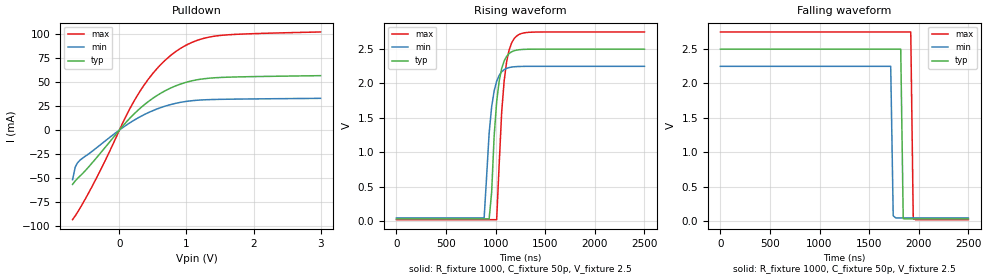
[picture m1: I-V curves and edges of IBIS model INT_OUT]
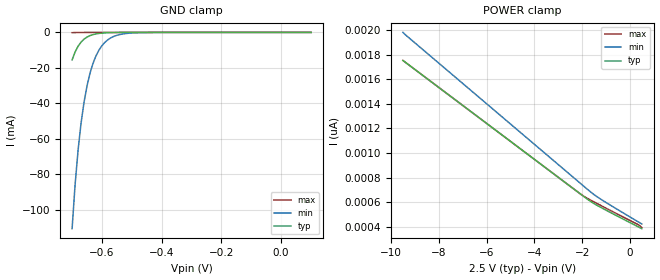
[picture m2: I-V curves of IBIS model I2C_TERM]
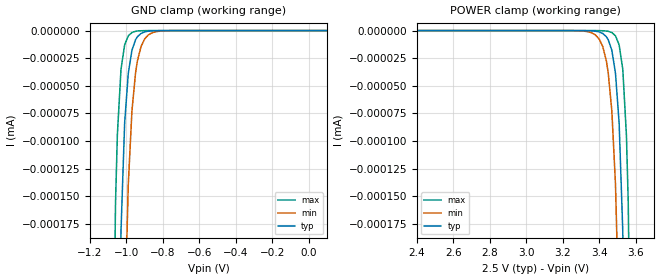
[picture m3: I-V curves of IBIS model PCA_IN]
|   NXP Semiconductors Inc.
|   Specialty Logic Products Group
|   IBIS model of PCA9544A
|   4-Channel I2C switch with
|   interrupt logic
[IBIS Ver]   3.2
[Comment Char]   |_char
| VDD typ = 2.5V, min = 2.25V and max = 2.75V
[File name]   pca9544a_2_5v.ibs
[File Rev]   1.0
[Date]   Nov 29, 2007 11:15:22 AM
[Source]
Generated by Seshadri Venkataramanan with IbisToolKit at Tempe, AZ
[Notes]
[Disclaimer]
* All rights reserved
NXP Semiconductors warrants and represents that the IBIS models identified
herein are owned by NXP Semiconductors (NXP). The
models provided are not warranted as fully representing all of the operating
characteristics and specifications of the semiconductor products to which the
models relate. Moreover, unless there is a
signed, written agreement to the contrary, these models are furnished on an "as
is" basis without support or warranty of any kind, either expressed or implied,
regarding the use thereof, and NXP specifically disclaims all implied warranties
of merchantability and
fitness of the models for any purpose.
NXP does not assume any liability arising out of the application or use of these
IBIS models including infringement of patents and
copyrights, nor does NXP convey any license under its patents and copyrights or
the rights of others.
NXP provides IBIS models as a service to our customers. You and your company
shall not distribute, convey, sell, or give these models
to anyone else without receiving prior written permission from NXP.(C) Copyright
2007 NXP Semiconductors
NXP Semiconductors (NXP) does not warrant that this model and any other
accompanying information (Model) accurately or fully represents the
operating characteristics and specifications of the semiconductor
products to which the Model relates.  Moreover, the Model is furnished
on an "as is" and with "all faults" basis, and without support or
warranty of any kind.  NXP disclaims all warranties, whether expressed
or implied or statutory, including without limitation all implied
warranties of non-infringement, merchantability and fitness for any
purpose, and those arising from a course of dealing or usage of trade.
NXP does not convey any license under its or any third party's patents,
copyrights or other intellectual property or proprietary rights.
You and your company assume any and all risks and liability arising out
of the application or use of the Model.
In no event shall NXP be liable for any direct, indirect, special,
consequential or incidental damages, however caused, whether in
warranty, contract or tort (including negligence), strict liability or
other legal theory, including, without limitation, for lost profits,
business interruption, or corruption or loss of data or information,
arising out of or in connection with the use of or the inability to use
the Model, even if NXP has been advised of the possibility of such
damages.
NXP provides the Model as a courtesy to our customers. You and your
company shall not distribute, convey, sell, or give the Model to anyone
else without receiving prior written permission from NXP.
NXP reserves the right to make changes without notice to the Model to
improve reliability, function, or design.
Please be aware that your receipt and subsequent use of the Model shall
serve as acceptance of these terms and conditions.  If you do not
accept these terms, return or destroy the Model immediately.
[Copyright]
2007
[Component]   PCA9544AD
Si_location Pin
Timing_location Pin
[Manufacturer]   NXP Semiconductors
[Package]
|   variable   typ   min   max
R_pkg   5.95E-02   5.36E-02   6.59E-02
L_pkg   4.21E-09   3.07E-09   5.91E-09
C_pkg   0.910E-12   0.758E-12   1.110E-12
|   SO20
[Pin] signal_name   model_name   R_pin   L_pin   C_pin
1   A0   PCA_IN   5.75E-02  5.91E-09  1.050E-12
2   A1   PCA_IN   6.25E-02  4.85E-09  1.040E-12
3   a2   PCA_IN   6.59E-02  3.92E-09  0.861E-12
4   INT0B   INT_IN   5.79E-02  3.32E-09  0.803E-12
5   SD0   I2C_TERM   5.36E-02  3.07E-09  0.758E-12
6   SC0   I2C_TERM   5.36E-02  3.07E-09  0.758E-12
7   INT1B   INT_IN   5.79E-02  3.32E-09  0.803E-12
8   SD1   I2C_TERM   6.59E-02  3.92E-09  0.861E-12
9   SC1   I2C_TERM   6.25E-02  4.85E-09  1.040E-12
10   Vss   GND   5.75E-02  5.91E-09  1.110E-12
11   INT2B   INT_IN   5.75E-02  5.91E-09  1.110E-12
12   SD2   I2C_TERM   6.25E-02  4.85E-09  1.040E-12
13   SC2   I2C_TERM   6.59E-02  3.92E-09  0.861E-12
14   INT3B   INT_IN   5.79E-02  3.32E-09  0.803E-12
15   SD3   I2C_TERM   5.36E-02  3.07E-09  0.758E-12
16   SC3   I2C_TERM   5.36E-02  3.07E-09  0.758E-12
17   INTB   INT_OUT   5.79E-02  3.32E-09  0.803E-12
18   SCL   I2C_TERM   6.59E-02  3.92E-09  0.861E-12
19   SDA   I2C_TERM   6.25E-02  4.85E-09  1.040E-12
20   Vdd   POWER   5.75E-02  5.91E-09  1.110E-12
[Component]   PCA9544APW
Si_location Pin
Timing_location Pin
[Manufacturer]   NXP Semiconductors
[Package]
|   variable   typ   min   max
R_pkg   7.24E-02   6.63E-02   8.34E-02
L_pkg   2.47E-09   2.09E-09   3.18E-09
C_pkg   0.341E-12   0.282E-12   0.420E-12
|   TSSOP20
[Pin] signal_name   model_name   R_pin   L_pin   C_pin
1   A0   PCA_IN   6.63E-02  3.18E-09  0.408E-12
2   A1   PCA_IN   6.67E-02  2.55E-09  0.398E-12
3   A2   PCA_IN   8.34E-02  2.35E-09  0.317E-12
4   INT0B   INT_IN   7.44E-02  2.16E-09  0.293E-12
5   SD0   I2C_TERM   7.10E-02  2.09E-09  0.282E-12
6   SC0   I2C_TERM   7.10E-02  2.09E-09  0.282E-12
7   INT1B   INT_IN   7.44E-02  2.16E-09  0.293E-12
8   SD1   I2C_TERM   8.34E-02  2.35E-09  0.317E-12
9   SC1   I2C_TERM   6.67E-02  2.55E-09  0.397E-12
10   Vss   GND   6.63E-02  3.18E-09  0.420E-12
11   INT2B   INT_IN   6.63E-02  3.17E-09  0.420E-12
12   SD2   I2C_TERM   6.67E-02  2.55E-09  0.397E-12
13   SC2   I2C_TERM   8.34E-02  2.35E-09  0.317E-12
14   INT3B   INT_IN   7.44E-02  2.16E-09  0.293E-12
15   SD3   I2C_TERM   7.10E-02  2.09E-09  0.282E-12
16   SC3   I2C_TERM   7.10E-02  2.09E-09  0.282E-12
17   INTB   INT_OUT   7.44E-02  2.16E-09  0.293E-12
18   SCL   I2C_TERM   8.34E-02  2.35E-09  0.317E-12
19   SDA   I2C_TERM   6.67E-02  2.55E-09  0.398E-12
20   Vdd   POWER   6.63E-02  3.17E-09  0.420E-12
[Component]   PCA9544ABS
Si_location Pin
Timing_location Pin
[Manufacturer]   NXP Semiconductors
[Package]
|   variable   typ   min   max
R_pkg   0.364   0.215   0.513
L_pkg   1.49E-09   1.04E-09   1.93E-09
C_pkg   0.149E-12   0.124E-12   0.173E-12
|   HVQFN20
[Package Model]   hvqfn20
[Pin] signal_name   model_name
1   A2   PCA_IN
2   INT0B   INT_IN
3   SD0   I2C_TERM
4   SC0   I2C_TERM
5   INT1B   INT_IN
6   SD1   I2C_TERM
7   SC1   I2C_TERM
8   Vss   GND
9   INT2B   INT_IN
10   SD2   I2C_TERM
11   SC2   I2C_TERM
12   INT3B   INT_IN
13   SD3   I2C_TERM
14   SC3   I2C_TERM
15   INTB   INT_OUT
16   SCL   I2C_TERM
17   SDA   I2C_TERM
18   Vdd   POWER
19   A0   PCA_IN
20   A1   PCA_IN
[Series Pin Mapping] pin_2 model_name   function_table_group
18   6   PCA_SW   1
18   9   PCA_SW   2
18   13   PCA_SW   3
18   16   PCA_SW   4
19   5   PCA_SW   1
19   8   PCA_SW   2
19   12   PCA_SW   3
19   15   PCA_SW   4
[Series Switch Groups]
|   Function Group States
|  default
Off 1 2 3 4 /
On 1 /
On 2 /
On 3 /
On 4 /
|  [Define Package Model]  MLF20_PCA9564.pkg
[Define Package Model]   hvqfn20
[Manufacturer]   Unknown
[OEM]   Unknown
[Description]   none
[Number of Pins]   20
[Pin Numbers]
|   1 = D2
1
|   2 = D3
2
|   3 = D4
3
|   4 = D5
4
|   5 = D6
5
|   6 = D7
6
|   7 = NC
7
|   8 = Vss
8
|   9 = WRn
9
|   10 = RDn
10
|   11 = CEn
11
|   12 = A0
12
|   13 = A1
13
|   14 = INTn
14
|   15 = RESETn
15
|   16 = SCL
16
|   17 = SDA
17
|   18 = Vdd
18
|   19 = D0
19
|   20 = D1
20
[Model Data]
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[End Model Data]
[End Package Model]
[Model]   PCA_SW
Model_type Series_switch
C_comp   0   0   0
[Temperature Range] 27   85   -40
[Voltage Range]   2.5   2.25   2.75
[On]
[R Series]   11   5   30
[C Series]   3p   NA   5p
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[Off]
|   variable   R(typ)   R(min)   R(max)
[R Series]   1e06   1e06   1e06
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| Models and submodels in the file (5): INT_OUT (Open_drain), I2C_TERM (Terminator), PCA_IN (Input), INT_IN (Input), PCA_SW (Series_switch)
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[Model]   INT_OUT
Model_type Open_drain
Vref=2.5
Vmeas=1.25
Rref=1000
Cref=1p
C_comp   2.2p   2p   2.3p
[Model Spec]
Vmeas   1.25   1.125   1.375
[Temperature Range] 27   85   -40
[Voltage Range]   2.5   2.25   2.75
[Pullup Reference]  2.5   2.25   2.75
[Pulldown Reference]0   0   0
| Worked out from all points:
|   slope of the pulldown table from 0 to 0.375 V, typ, clamps not added: 14.1 ohm
|   falling waveform, R_fixture 1000, C_fixture 50p, V_fixture 2.5: 20-80 % time 15.2ns typ, 15.4ns min, 15.2ns max; typ from 2.5 V to 0.029 V
|   rising waveform, R_fixture 1000, C_fixture 50p, V_fixture 2.5: 20-80 % time 70ns typ, 73.5ns min, 73.2ns max; typ from 0.029 V to 2.5 V
[Pulldown]
-700mV    -56.73mA   -51.78mA   -93.46mA
-660mV    -53.03mA   -38.68mA   -89.46mA
-590mV    -48.07mA   -31.52mA   -81.6mA
-330mV    -27.89mA   -17.91mA   -48.27mA
80mV      6.56mA     3.993mA    11.93mA
270mV     20.17mA    12.32mA    36.31mA
380mV     26.83mA    16.38mA    48.06mA
530mV     34.54mA    21.07mA    61.59mA
790mV     44.53mA    26.96mA    79.11mA
1.09V     51.37mA    30.57mA    91.51mA
1.43V     54.44mA    31.82mA    97.86mA
3V        56.6mA     32.97mA    102.1mA
[Falling Waveform]
R_fixture=1000
C_fixture=50p
V_fixture=2.5
V_fixture_min=2.25
V_fixture_max=2.75
0s        2.5V       2.25V      2.75V
1.717us   2.5V       2.25V      2.75V
1.742us   2.5V       74.23mV    2.75V
1.768us   2.5V       43.95mV    2.75V
1.818us   2.5V       43.54mV    2.75V
1.843us   33.16mV    43.55mV    2.75V
1.919us   29.47mV    43.54mV    2.75V
1.944us   29.47mV    43.54mV    33.07mV
1.97us    29.47mV    43.54mV    17.77mV
2.5us     29.47mV    43.54mV    17.77mV
[Rising Waveform]
R_fixture=1000
C_fixture=50p
V_fixture=2.5
V_fixture_min=2.25
V_fixture_max=2.75
0s        29.47mV    43.53mV    17.78mV
883.8ns   29.48mV    43.54mV    17.78mV
934.3ns   29.48mV    1.279V     17.78mV
959.6ns   417.2mV    1.661V     17.79mV
1.01us    1.733V     2.033V     17.8mV
1.061us   2.218V     2.17V      1.58V
1.086us   2.329V     2.202V     2.041V
1.136us   2.437V     2.232V     2.49V
1.212us   2.486V     2.246V     2.692V
2.5us     2.5V       2.25V      2.75V
[Ramp]
R_load=1000
dV/dt_r   1.482E+0/1.015E-9   1.471E+0/1.420E-9   1.490E+0/1.159E-9
dV/dt_f   1.482E+0/1.288E-9   1.471E+0/2.101E-9   1.490E+0/6.639E-10
|[End   INT_OUT
| [End   INT_OUT
|  [End   INT_OUT
[Model]   I2C_TERM
Model_type Terminator
C_comp   1.7p   1.7p   1.7p
[Temperature Range] 27   85   -40
[Voltage Range]   2.5   2.25   2.75
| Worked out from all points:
|   GND clamp passes 1 mA (typ) near -0.62 V on its own axis
[GND Clamp]
|   -6.000000E-1   -1.554225E-1   -1.242642E-1   -2.666059E-1
|   -5.000000E-1   -1.602113E-1   -1.179351E-1   -2.662641E-1
|   -4.000000E-1   -1.574088E-1   -1.099432E-1   -2.800035E-1
-700mV    -15.49mA   -110.5mA   -166uA
-690mV    -11.04mA   -85.85mA   -101uA
-680mV    -7.802mA   -66.38mA   -61.45uA
-670mV    -5.469mA   -51.14mA   -37.37uA
-660mV    -3.806mA   -39.28mA   -22.72uA
-650mV    -2.632mA   -30.08mA   -13.81uA
-640mV    -1.812mA   -22.97mA   -8.398uA
-620mV    -849.6uA   -13.22mA   -3.104uA
-580mV    -183uA     -4.119mA   -424nA
-540mV    -39.08uA   -1.192mA   -57.99nA
-480mV    -3.844uA   -174.3uA   -3.016nA
100mV     19.7pA     22.78pA    19.7pA
[POWER Clamp]
-9.5V     1.752nA    1.98nA     1.752nA
-2.03V    661.4pA    746.5pA    661.8pA
-1.62V    603.2pA    679.7pA    614.9pA
-1.32V    568.9pA    637.6pA    584.1pA
300mV     405pA      446.1pA    422.3pA
500mV     385.1pA    423.1pA    394pA
[Model]   PCA_IN
Model_type Input
Vinh=1.7
Vinl=0.5
C_comp   0.5p   0.5p   0.5p
[Model Spec]
[Temperature Range] 27   85   -40
[Voltage Range]   2.5   2.25   2.75
[POWER Clamp Reference]2.5   2.25   2.75
[GND Clamp Reference]0   0   0
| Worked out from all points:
|   GND clamp passes 1 mA (typ) near -1.25 V on its own axis
[GND Clamp]
-1.7V     -4.583A    -3.655A    -5.795A
-1.08V    -1.254uA   -2.572uA   -421.3nA
-1.06V    -578.9nA   -1.345uA   -155.7nA
-1.05V    -393.3nA   -972.8nA   -94.64nA
-1.03V    -181.5nA   -508.9nA   -34.97nA
-1.01V    -83.76nA   -266.2nA   -12.93nA
-990mV    -38.66nA   -139.2nA   -4.777nA
-970mV    -17.84nA   -72.82nA   -1.766nA
-950mV    -8.234nA   -38.09nA   -653.2pA
-920mV    -2.582nA   -14.41nA   -147.4pA
-860mV    -254.6pA   -2.063nA   -8.255pA
100mV     100fA      100fA      100fA
[POWER Clamp]
2.4V      100fA      100fA      100fA
3.36V     -254.6pA   -2.063nA   -8.255pA
3.42V     -2.582nA   -14.41nA   -147.4pA
3.45V     -8.234nA   -38.09nA   -653.2pA
3.47V     -17.84nA   -72.82nA   -1.766nA
3.49V     -38.66nA   -139.2nA   -4.777nA
3.51V     -83.76nA   -266.2nA   -12.93nA
3.53V     -181.5nA   -508.9nA   -34.97nA
3.55V     -393.3nA   -972.8nA   -94.64nA
3.56V     -578.9nA   -1.345uA   -155.7nA
3.58V     -1.254uA   -2.572uA   -421.3nA
4.2V      -4.583A    -3.655A    -5.795A
